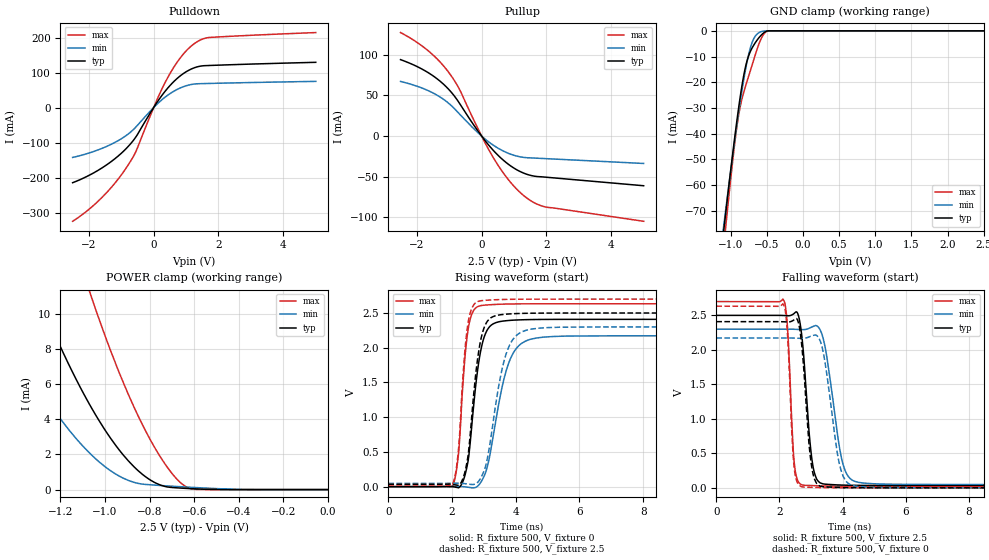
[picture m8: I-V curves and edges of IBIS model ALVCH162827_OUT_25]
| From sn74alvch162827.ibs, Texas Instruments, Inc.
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[Model]   ALVCH162827_OUT_25
Model_type  3-state
Enable   Active-Low
Vref =   0
Rref =   500
Cref =   30p
Vmeas =   1.25
| variable   typ   min   max
C_comp   7.36pF   6.47pF   8.47pF
| C_pullup   8.54pF   7.05pF   9.38pF
| C_pulldown   11.88pF   9.05pF   15.56pF
| C_tri-state   7.36pF   6.47pF   8.47pF
[Temperature Range]   40   100   -40
| Ambient temperature   25   85   -40
[Voltage range]   2.5   2.3   2.7
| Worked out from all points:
|   slope of the pulldown table from 0 to 0.375 V, typ, clamps not added: 7.66 ohm
|   slope of the pullup table from 0 to 0.375 V, typ, clamps not added: 20.6 ohm
|   GND clamp passes 1 mA (typ) near -0.55 V on its own axis
|   POWER clamp passes 1 mA (typ) near -0.84 V on its own axis
|   rising waveform, R_fixture 500, V_fixture 0: 20-80 % time 352ps typ, 568ps min, 246ps max; typ from 0 V to 2.41 V
|   falling waveform, R_fixture 500, V_fixture 2.5: 20-80 % time 248ps typ, 420ps min, 160ps max; typ from 2.5 V to 0.034 V
|   rising waveform, R_fixture 500, V_fixture 2.5: 20-80 % time 334ps typ, 512ps min, 241ps max; typ from 0.034 V to 2.5 V
|   falling waveform, R_fixture 500, V_fixture 0: 20-80 % time 237ps typ, 389ps min, 155ps max; typ from 2.41 V to 0 V
[GND Clamp]
| ALVCH162827_OUT_25
|   Voltage   I(typ)   I(min)   I(max)
-2.5V     -467.6mA   -428.1mA   -528.9mA
-1.095V   -77.15mA   -75.2mA    -83.44mA
-1.08V    -73.42mA   -71.82mA   -79.21mA
-1.06V    -68.5mA    -67.35mA   -73.63mA
-920mV    -36.01mA   -37.55mA   -38.35mA
-870mV    -25.87mA   -27.84mA   -29.62mA
-815mV    -16.6mA    -18.16mA   -23.39mA
-770mV    -11.23mA   -11.42mA   -19.2mA
-710mV    -6.971mA   -4.944mA   -13.82mA
-595mV    -2.192mA   -484.1uA   -4.058mA
-480mV    -19.21uA   -57.93uA   -14.88uA
2.5V      83.8pA     43.75nA    39.19pA
[POWER Clamp]
| ALVCH162827_OUT_25
|   Voltage   I(typ)   I(min)   I(max)
-2.5V     62.78mA    42.4mA     93.4mA
-1.535V   19.08mA    11.24mA    32.91mA
-1.515V   18.34mA    10.73mA    31.84mA
-1.295V   10.9mA     5.78mA     20.85mA
-1.165V   7.185mA    3.45mA     15.09mA
-1.06V    4.638mA    1.967mA    10.93mA
-950mV    2.483mA    868.5uA    7.093mA
-845mV    1.005mA    337.3uA    4.026mA
-745mV    230.8uA    229.2uA    1.729mA
-655mV    82.47uA    160.2uA    326.5uA
-600mV    45.53uA    121.2uA    16.21uA
-31.15fV  83.8pA     317.5pA    46.7pA
[Pulldown]
| ALVCH162827_OUT_25
|   Voltage   I(typ)   I(min)   I(max)
-2.5V     -214.5mA   -142.4mA   -324.7mA
-1.625V   -174.1mA   -117.7mA   -259.4mA
-1.225V   -148.2mA   -100.9mA   -219.1mA
-870mV    -119.2mA   -81.23mA   -175.5mA
-550mV    -84.06mA   -55.7mA    -125.8mA
75mV      10.83mA    7.022mA    16.48mA
430mV     55.09mA    35.04mA    84.84mA
820mV     90.47mA    55.98mA    141.7mA
1.215V    112.2mA    66.71mA    179.9mA
1.465V    118.6mA    68.28mA    193.9mA
1.72V     120.2mA    68.88mA    200.2mA
5V        129.2mA    74.77mA    214.1mA
[Pullup]
| ALVCH162827_OUT_25
|   Voltage   I(typ)   I(min)   I(max)
-2.5V     93.89mA    67.09mA    127.2mA
-1.675V   78.56mA    56.27mA    105.7mA
-1.335V   69.15mA    49.28mA    93.27mA
-1.035V   58.23mA    40.89mA    79.35mA
-685mV    40.38mA    27.22mA    57.59mA
15mV      -812.9uA   -531.7uA   -1.2mA
420mV     -20.15mA   -12.8mA    -30.36mA
885mV     -36.42mA   -22.17mA   -56.52mA
1.355V    -46.47mA   -26.53mA   -75.01mA
1.67V     -49.6mA    -27.19mA   -82.95mA
1.985V    -50.63mA   -27.82mA   -87.32mA
5V        -61.14mA   -33.76mA   -104.8mA
[Ramp]
| ALVCH162827_OUT_25
| variable   typ   min   max
dV/dt_r   1.46/3.60E-10   1.31/5.75E-10   1.58/2.54E-10
dV/dt_f   1.51/2.61E-10   1.38/4.35E-10   1.63/1.66E-10
R_load = 500
[Rising Waveform]
| ALVCH162827_OUT_25
R_fixture =   500
C_fixture =   0
L_fixture =   0
V_fixture =   0
V_fixture_min = 0
V_fixture_max = 0
|   Time   V(typ)   V(min)   V(max)
0s        334.1pV    1.357nV    238.1pV
2.015ns   -365.3uV   2.229mV    8.729mV
2.205ns   -16.04mV   3.099mV    482.7mV
2.395ns   146.9mV    -2.72mV    1.805V
2.52ns    420.6mV    -10.02mV   2.305V
2.785ns   1.615V     172.6uV    2.587V
2.995ns   2.135V     140.2mV    2.612V
3.825ns   2.394V     1.833V     2.63V
4.87ns    2.408V     2.153V     2.633V
50ns      2.409V     2.172V     2.633V
[Falling Waveform]
| ALVCH162827_OUT_25
R_fixture =   500
C_fixture =   0
L_fixture =   0
V_fixture =   2.5
V_fixture_min = 2.3
V_fixture_max = 2.7
|   Time   V(typ)   V(min)   V(max)
0s        2.5V       2.3V       2.7V
2.14ns    2.498V     2.3V       2.715V
2.26ns    2.495V     2.3V       2.29V
2.48ns    2.534V     2.298V     317.1mV
2.795ns   1.751V     2.294V     37.07mV
2.995ns   541.5mV    2.324V     33.77mV
3.18ns    126.7mV    2.349V     30.61mV
4.025ns   39.89mV    323.9mV    24.95mV
4.675ns   35.35mV    68.96mV    24.24mV
50ns      33.7mV     47.62mV    23.99mV
[Rising Waveform]
| ALVCH162827_OUT_25
R_fixture =   500
C_fixture =   0
L_fixture =   0
V_fixture =   2.5
V_fixture_min = 2.3
V_fixture_max = 2.7
|   Time   V(typ)   V(min)   V(max)
0s        33.7mV     47.62mV    23.99mV
2.015ns   32.32mV    49.51mV    33.71mV
2.2ns     18.49mV    49.46mV    523.2mV
2.375ns   162.7mV    43.94mV    1.788V
2.495ns   422.8mV    37.97mV    2.331V
2.745ns   1.626V     40.13mV    2.647V
2.92ns    2.151V     140mV      2.677V
3.735ns   2.485V     1.958V     2.696V
4.685ns   2.498V     2.28V      2.7V
50ns      2.5V       2.3V       2.7V
[Falling Waveform]
| ALVCH162827_OUT_25
R_fixture =   500
C_fixture =   0
L_fixture =   0
V_fixture =   0
V_fixture_min = 0
V_fixture_max = 0
|   Time   V(typ)   V(min)   V(max)
0s        2.409V     2.172V     2.633V
2.135ns   2.407V     2.172V     2.649V
2.25ns    2.405V     2.172V     2.266V
2.465ns   2.436V     2.171V     299.4mV
2.725ns   1.977V     2.167V     14.15mV
3.11ns    128.3mV    2.214V     6.45mV
3.39ns    15.64mV    1.96V      3.271mV
3.94ns    5.46mV     272.4mV    937.9uV
4.51ns    1.618mV    18.09mV    281.1uV
50ns      2.234nV    -3.007nV   -1.121nV
